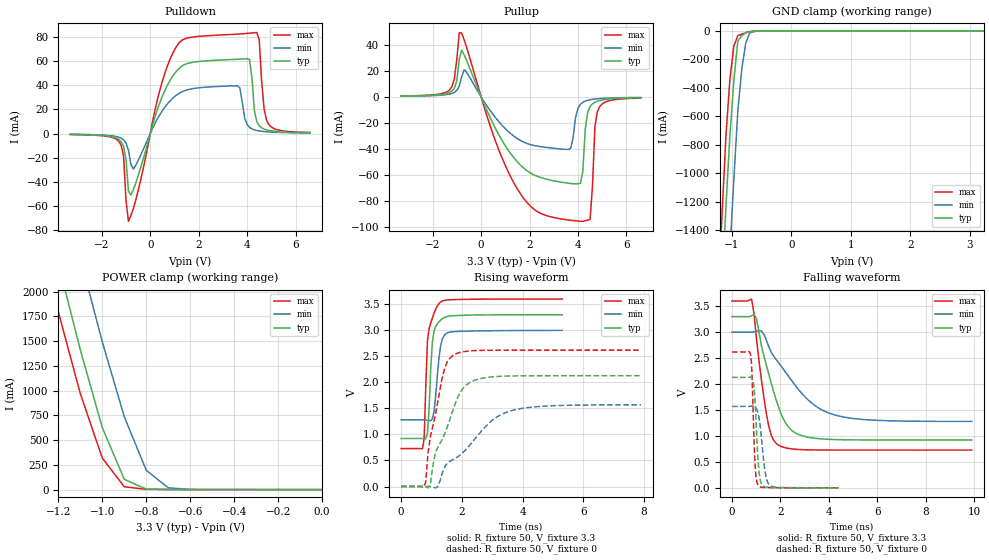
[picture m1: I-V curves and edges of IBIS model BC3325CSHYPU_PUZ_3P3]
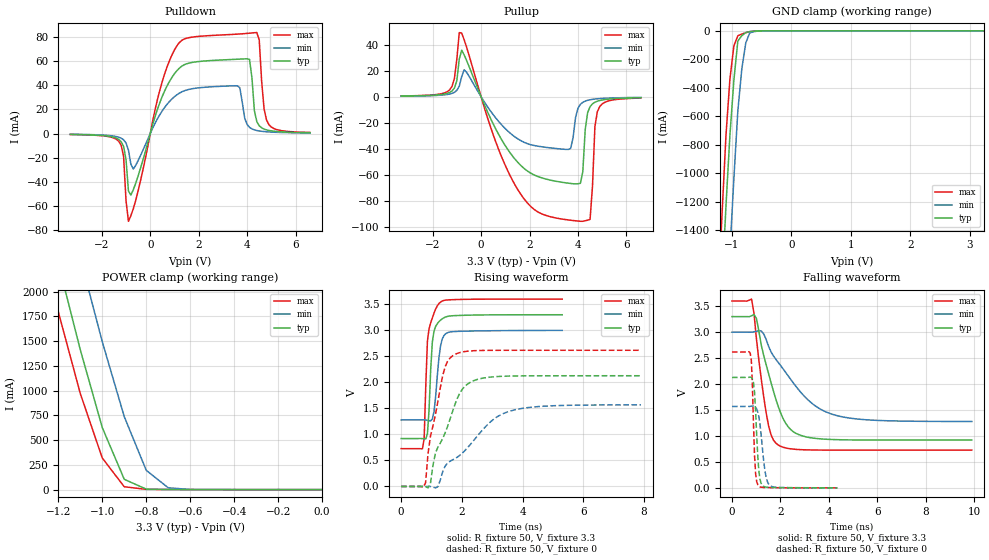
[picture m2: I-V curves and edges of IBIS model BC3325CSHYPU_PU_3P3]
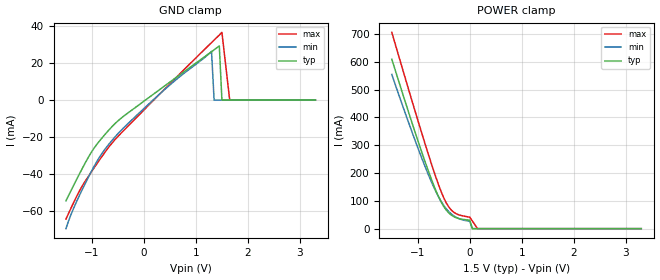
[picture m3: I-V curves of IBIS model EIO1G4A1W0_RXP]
[IBIS ver]   4.1
[File name]   xio3130_sandeer.ibs
[File Rev]   1.0
[Date]   September 10, 2007
[Source]   TI
[Notes]   Ver 1.1: Original September 10, 2007
| REV LOG:   1.0 original on August 21, 2006
|   Ver 1.1 is IBIS for PG 2.
[Disclaimer] Please be aware that in the absence of a written agreement
   Texas Instruments(TI) assumes no liability for: (1) The
   accuracy of the IBIS models provided to your company (2) The
   proper functioning of these Models in your design or for any
   resulting applications;or (3) Infringement of
   patents,copyrights or intellectual property rights resulting
   from your use of these models. TI provides IBIS Models as a
   service to our customers and therefore reserves the right to
   limit distribution of the Models.
[Copyright]   Property of Texas Instruments Incorporated. Unauthorised
   reproduction and/or distribution is strictly prohibited. This
   product is protected under copyright law and trade secret law
   as an unpublished work. Created 2007,(C) Copyright 2007,
   Texas Instruments Incorporated., All Rights Reserved. These
   commodities are under the U.S. Government distribution license
   control.As such,they are not to be re-exported without the
   prior approval of the U.S. Department of Commerce.
|   Component XIO3130
[Component]   XIO3130
[Manufacturer]   Texas Instruments.
[Package]
| variable   typ   min   max
R_pkg   2.09305e-001  8.11042e-003  5.46728e-001
L_pkg   3.90785e-009  1.26190e-009  1.07040e-008
C_pkg   1.04479e-012  5.09606e-013  6.63618e-012
[Pin]  signal_name   model_name  R_pin   L_pin   C_pin
A1 	PERST2		BC3325CSHYPU 	3.48182e-01	6.76130e-09	1.52376e-12
A12 	 PWR_GD0_GPIO2	BC3325CSHYPU 	3.39794e-01	4.78530e-09	6.39971e-13
A13 	VPP_1		POWER   2.77158e-01	4.95020e-09	1.35433e-12
A14	GPIO12		BC3325CSHYPU 	3.17830e-01	5.67010e-09	1.12048e-12
A2	PERST1		BC3325CSHYPU 	3.16708e-01	5.94340e-09	1.37649e-12
A6	DN_PERP_0	EIO1G4A1W0_RXP	3.07358e-01	4.42330e-09	9.38426e-13
A8	DN_PETP_0	EIO1G4A1W0_TX	3.02145e-01	4.33380e-09	1.15943e-12
A9	REFCKOP_0	 REFCLKOUT_C	3.39864e-01	4.83750e-09	9.84588e-13
B1 	PERST		IC33SFSHYPD	2.86998e-01	5.02970e-09	1.46470e-12
B11	PWR_ON0_GPIO1	BC3325CSHYPU 	2.96203e-01	3.82290e-09	6.38354e-13
B12	VPP_2		POWER   2.28630e-01	3.58240e-09	1.23695e-12
B13	GPIO13		BC3325CSHYPU 	2.56386e-01	4.03580e-09	1.36016e-12
B14	SCL		BC3325CSHYPU 	3.81111e-01	5.90920e-09	9.17494e-13
B5 	PERST0		BC3325CSHYPU 	2.52744e-01	3.39930e-09	9.88828e-13
B6	DN_PERN_0	EIO1G4A1W0_RXN	2.97653e-01	4.07660e-09	9.46291e-13
B8	DN_PETN_0	EIO1G4A1W0_TX	2.99772e-01	4.12360e-09	1.05127e-12
B9	REFCKON_0	REFCLKOUT_C	3.37041e-01	4.54020e-09	1.18566e-12
C10	DPSTRP0		BC3325CSHYPU 	1.67776e-01	2.10160e-09	8.80891e-13
C12	GPIO3		BC3325CSHYPU 	2.02085e-01	2.62660e-09	1.12832e-12
C2	GRST		IC33THYPU	2.55732e-01	3.73630e-09	1.72787e-12
C3	WAKE		BC3350BTOD	2.04369e-01	2.88420e-09	1.47207e-12
C4	VREG_EN   NC   1.72568e-01	2.16550e-09	1.53275e-12
C6	PRSNT0_GPIO0	BC3325CSHYPU 	1.59277e-01	2.01830e-09	1.29989e-12
D1	VSSDREF   GND   2.96673e-01	4.40840e-09	6.56277e-13
D13	SDA		BC3325CSHYPU 	3.10044e-01	4.05030e-09	8.29410e-13
D14	PRSNT1_GPIO4	BC3325CSHYPU 	2.72028e-01	4.51280e-09	8.91943e-13
D2	REFR0		NC   2.08243e-01	3.12100e-09	8.72610e-13
D4	TM_EN		IC33S   1.71885e-01	1.87770e-09	1.56170e-12
E1	VAUX33REF	POWER   2.95994e-01	4.32000e-09	5.85849e-13
E2	VDD33REF	POWER   2.58088e-01	3.37240e-09	7.27540e-13
E3	REFR1		NC   1.65373e-01	2.05030e-09	9.51770e-13
E4	VSSAREF	GND	1.71892e-01	1.87280e-09	1.13752e-12
F13	DN_PERP_1	EIO1G4A1W0_RXP	3.39229e-01	4.52580e-09	1.00466e-12
F14	DN_PERN_1	EIO1G4A1W0_RXP	3.40188e-01	4.70740e-09	8.48746e-13
F3	VDDAREF   POWER   1.96308e-01	2.26680e-09	1.07035e-12
G1	UP_PETP_1	EIO1G4A1W0_TX	2.92665e-01	4.25920e-09	7.86997e-13
G2	UP_PETN_1	EIO1G4A1W0_TX	2.89056e-01	4.03470e-09	9.71695e-13
H13	DN_PETP_1	EIO1G4A1W0_TX	2.91932e-01	3.96270e-09	8.44904e-13
H14	DN_PETN_1	EIO1G4A1W0_TX	2.91177e-01	4.24470e-09	8.54606e-13
J1 	 UP_PERP_1	EIO1G4A1W0_RXP	3.39760e-01	4.81770e-09	9.53436e-13
J14	REFCKON_1	REFCLKOUT_C	3.28820e-01	4.73900e-09	8.56505e-13
J2	 UP_PERN_1	EIO1G4A1W0_RXN	3.40049e-01	4.64620e-09	1.07197e-12
K14	REFCKOP_1	REFCLKOUT_C	3.31929e-01	4.68100e-09	6.52614e-13
L1	REFCKIP_1	PCIEREFIN_V30	3.97574e-01	6.00690e-09	1.41140e-12
L12	 PWR_ON1_GPIO5	BC3325CSHYPU 	1.85893e-01	2.41880e-09	1.02367e-12
L13	DPSTRP1		BC3325CSHYPU 	3.04921e-01	3.99150e-09	9.55643e-13
L2	REFCKIN_1	PCIEREFIN_V30	3.95837e-01	5.85920e-09	1.39246e-12
L3	GPIO18		BC3325CSHYPU 	2.29605e-01	3.05390e-09	1.35688e-12
M10	PRSNT2_GPIO8	BC3325CSHYPU 	1.74120e-01	2.17390e-09	1.07131e-12
M13	PWR_GD1_GPIO6	BC3325CSHYPU 	2.33053e-01	3.57840e-09	1.07590e-12
M14	GPIO15		BC3325CSHYPU 	2.77478e-01	4.66060e-09	8.47070e-13
M3	GPIO17_PWR_OVER	BC3325CSHYPU 	1.98049e-01	2.79690e-09	1.22160e-12
N11	GPIO11		BC3325CSHYPU 	2.23391e-01	3.27840e-09	8.83452e-13
N12	GPIO14		BC3325CSHYPU 	2.29447e-01	3.59270e-09	7.28550e-13
N2	CLKREQ_UP	BC3350BTOD	2.94360e-01	4.68110e-09	1.18772e-12
N3 	PWR_ON2_GPIO9	BC3325CSHYPU 	3.25542e-01	4.54360e-09	9.29756e-13
N4	DPSTRP2		BC3325CSHYPU 	3.06995e-01	4.01710e-09	7.83007e-13
N7	DN_PETP_2	EIO1G4A1W0_TX	2.90192e-01	3.96320e-09	9.35839e-13
N9	DN_PERP_2	EIO1G4A1W0_RXP	3.30597e-01	4.43580e-09	1.08021e-12
P1	REFCLK_SEL	IC33S   3.11848e-01	5.57690e-09	1.10777e-12
P12	GPIO16		BC3325CSHYPU 	3.48550e-01	4.99450e-09	8.65165e-13
P13	GPIO7		BC3325CSHYPU 	3.71036e-01	5.56470e-09	7.58018e-13
P2	PWR_GD2_GPIO10	BC3325CSHYPU 	2.86683e-01	5.10680e-09	1.31629e-12
P5	REFCKOP_2	 REFCLKOUT_C	3.43286e-01	4.84920e-09	5.90517e-13
P6	REFCKON_2	 REFCLKOUT_C	3.39679e-01	4.78910e-09	7.53869e-13
P7	DN_PETN_2	EIO1G4A1W0_TX	2.91402e-01	4.20940e-09	8.89549e-13
P9	DN_PERN_2	EIO1G4A1W0_RXN	3.35460e-01	4.62110e-09	9.64954e-13
[Model Selector]   BC3325CSHYPU
BC3325CSHYPU_PUZ_3P3  Cell operated at 3.3(nom) PULLUP_ON
BC3325CSHYPU_PU_3P3  Cell operated at 3.3(nom) PULLUP_OFF
[Model Selector]   IC33SFSHYPD
IC33SFSHYPD_3P3PD   Cell operated at VDDS=3.3V(typ) with pulldown "on"
IC33SFSHYPD_3P3PDZ   Cell operated at VDDS=3.3V(typ) with pulldown "off"
[Model Selector] IC33THYPU
IC33THYPU_3P3PU   Cell operated at VDDS=3.3V(nom) with Pullup "on"
IC33THYPU_3P3PUZ   Cell operated at VDDS=3.3V(nom) with Pullup "off"
[Model Selector]   IC33S
IC33S_2P5   Cell operated at VDDS=2.5V(nom)
IC33S_3P3   Cell operated at VDDS=3.3V(nom)
[Model] EIO1G4A1W0_TX
Model_type Output
Polarity Non-Inverting
Cref = 2.0pF
Rref = 50
Vref = 1.0V
Vmeas =1.0V
|   typ   min   max
C_comp   1.603pF   1.594pF   1.637pF
|[Model Spec]
[Driver Schedule]
| Model_name Rise_on_dly Rise_off_dly Fall_on_dly Fall_off_dly
high_high 0.0nS 0.4nS NA NA
medium_high 0.401nS 1.95nS NA NA
low_low NA NA 0.0nS 0.40nS
medium_low NA NA 0.401nS 2.05nS
[Temperature Range]   25   125   -40
[Voltage Range] 1.50V 1.35V 1.65V
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[Ramp]
| variable   typ   min   max
dV/dt_r 1V/0.001ns  0.21654V/0.0277367ns  0.198V/0.0212173ns
dV/dt_f 1V/0.001ns  0.21654V/0.0277367ns  0.198V/0.0212173ns
R_load = 50
| Models and submodels in the file (18): BC3325CSHYPU_PUZ_3P3 (I/O), BC3325CSHYPU_PU_3P3 (I/O), EIO1G4A1W0_RXP (Input), EIO1G4A1W0_RXN (Input), REFCLKOUT_C (Output), IC33SFSHYPD_3P3PD (Input), IC33SFSHYPD_3P3PDZ (Input), EIO1G4A1W0_TX (Output), high_high (Open_source), low_low (Open_drain), medium_high (Open_source), medium_low (Open_drain), IC33THYPU_3P3PU (Input), IC33THYPU_3P3PUZ (Input), BC3350BTOD (I/O_open_drain), IC33S_2P5 (Input), IC33S_3P3 (Input), PCIEREFIN_V30 (Input)
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|   Model Cell BC3325CSHYPU_PUZ_3P3
[Model]   BC3325CSHYPU_PUZ_3P3
Model_type   I/O
Polarity   Non-Inverting
Enable   Active-Low
Vinl =  0.8v
Vinh =  2v
Cref =  15.0000pF
Rref =  100.0000M
Vref =  0V
Vmeas =  1.65
C_comp   2.096801p   2.080601p   2.168299p
[Model Spec]
Vinl   0.8v   0.8V   0.8V
Vinh   2v   2V   2V
[Temperature Range]   25   125   -40
[Voltage Range]   3.3   3   3.6
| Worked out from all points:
|   slope of the pulldown table from 0 to 0.495 V, typ, clamps not added: 16.1 ohm
|   slope of the pullup table from 0 to 0.495 V, typ, clamps not added: 23.9 ohm
|   GND clamp passes 1 mA (typ) near -0.57 V on its own axis
|   POWER clamp passes 1 mA (typ) near -0.70 V on its own axis
|   rising waveform, R_fixture 50, V_fixture 3.3: 20-80 % time 131ps typ, 171ps min, 141ps max; typ from 0.923 V to 3.3 V
|   rising waveform, R_fixture 50, V_fixture 0: 20-80 % time 804ps typ, 1.58ns min, 487ps max; typ from 0.001 V to 2.13 V
|   falling waveform, R_fixture 50, V_fixture 3.3: 20-80 % time 871ps typ, 1.74ns min, 492ps max; typ from 3.3 V to 0.923 V
|   falling waveform, R_fixture 50, V_fixture 0: 20-80 % time 145ps typ, 222ps min, 111ps max; typ from 2.13 V to 0.001 V
[POWER_clamp]
|   voltage   I(typ)   I(min)   I(max)
-3.3V     22.69A     23.55A     22.21A
-1.233V   2.591A     3.534A     2.093A
-1.2V     2.287A     3.229A     1.795A
-1.167V   1.995A     2.933A     1.52A
-1.1V     1.413A     2.34A      970.4mA
-1.067V   1.151A     2.058A     753.2mA
-1.033V   888.5mA    1.776A     536.1mA
-1V       626.4mA    1.494A     318.9mA
-900mV    104mA      736.8mA    28.83mA
-800mV    4.946mA    194.9mA    2.696mA
-700mV    998.1uA    18.43mA    1.144mA
-11.55fV  218.9pA    3.023nA    211.8pA
[Pulldown]
|   voltage   I(typ)   I(min)   I(max)
-3.3V     -705.5uA   -563.9uA   -760.4uA
-1.3V     -4.855mA   -3.026mA   -6.366mA
-1.1V     -10.66mA   -5.175mA   -19.03mA
-900mV    -47.6mA    -13.63mA   -72.85mA
-700mV    -46.65mA   -29.39mA   -62.46mA
1.1V      52.19mA    32.2mA     72.89mA
3.6V      61.75mA    39.68mA    82.61mA
4.1V      61.59mA    5.155mA    83.39mA
4.4V      9.95mA     2.546mA    83.89mA
4.7V      3.744mA    1.667mA    20.57mA
4.9V      2.605mA    1.352mA    7.423mA
6.6V      709.5uA    512.8uA    930uA
[Pullup]
|   voltage   I(typ)   I(min)   I(max)
-3.3V     505.9uA    408uA      584.9uA
-1.3V     3.261mA    2.062mA    5.225mA
-800mV    35.78mA    15.51mA    48.94mA
600mV     -24.59mA   -16.18mA   -34.36mA
1.6V      -52.1mA    -33.35mA   -73.91mA
3.7V      -66.73mA   -39.75mA   -95mA
4.2V      -57.72mA   -4.291mA   -95.81mA
4.3V      -25.25mA   -3.364mA   -95.38mA
4.5V      -7.634mA   -2.331mA   -94.34mA
4.7V      -4.24mA    -1.775mA   -22.94mA
4.9V      -2.904mA   -1.43mA    -7.534mA
6.6V      -771.5uA   -533.2uA   -1.015mA
[GND_clamp]
|   voltage   I(typ)   I(min)   I(max)
-3.3V     -22.48A    -23.28A    -22.04A
-1.233V   -2.398A    -3.286A    -1.879A
-1.167V   -1.809A    -2.69A     -1.297A
-1.1V     -1.235A    -2.104A    -738.1mA
-1.033V   -735.2mA   -1.553A    -340.6mA
-966.7mV  -347.6mA   -1.039A    -106.1mA
-900mV    -71.93mA   -563.2mA   -34.66mA
-833.3mV  -34.38mA   -267.8mA   -23.1mA
-766.7mV  -12.31mA   -84.87mA   -13.47mA
-700mV    -5.7mA     -14.32mA   -5.752mA
-500mV    -215.1uA   -473.8uA   -210uA
3.233V    -4.928uA   12.61uA    -38.06uA
[Ramp]
| variable   typ   min   max
dV/dt_r   1.29409/0.8072212n  0.9574059/1.586115n   1.586195/0.4872986n
dV/dt_f   1.451701/0.8772609n   1.051893/1.749039n   1.750196/0.494297n
R_load = 50
[Rising Waveform]
R_fixture = 50
V_fixture = 3.3
V_fixture_min = 3
V_fixture_max = 3.6
|   time   V(typ)   V(min)   V(max)
0s        922.7mV    1.28V      729.2mV
703ps     921.8mV    1.281V     727mV
758ps     915.9mV    1.281V     919.8mV
866ps     1.014V     1.274V     2.793V
920ps     1.476V     1.265V     3.029V
1.028ns   2.771V     1.3V       3.237V
1.083ns   2.982V     1.438V     3.33V
1.299ns   3.196V     2.699V     3.544V
1.624ns   3.277V     2.968V     3.587V
5.308ns   3.3V       2.999V     3.6V
[Rising Waveform]
R_fixture = 50
V_fixture = 0
V_fixture_min = 0
V_fixture_max = 0
|   time   V(typ)   V(min)   V(max)
0s        1.034mV    901.2uV    1.259mV
805ps     -3.192mV   1.663mV    73.26mV
886ps     -25.74mV   2.498mV    638.9mV
966ps     62.2mV     -720.8uV   971.7mV
1.127ns   640.5mV    -25.36mV   1.378V
1.369ns   925.5mV    285.7mV    2.132V
1.772ns   1.576V     537.9mV    2.539V
2.336ns   2.02V      847.5mV    2.608V
3.545ns   2.123V     1.443V     2.618V
7.9ns     2.129V     1.569V     2.619V
[Falling Waveform]
R_fixture = 50
V_fixture = 3.3
V_fixture_min = 3
V_fixture_max = 3.6
|   time   V(typ)   V(min)   V(max)
0s        3.3V       3V         3.6V
807ps     3.315V     2.999V     3.636V
908ps     3.342V     3.006V     3.368V
1.009ns   3.263V     3.016V     2.878V
1.413ns   2.374V     2.857V     1.447V
1.615ns   2.028V     2.619V     1.024V
1.918ns   1.562V     2.414V     825.2mV
2.625ns   1.057V     1.967V     744.6mV
4.241ns   931.8mV    1.405V     729.5mV
9.896ns   922.7mV    1.281V     729.2mV
[Falling Waveform]
R_fixture = 50
V_fixture = 0
V_fixture_min = 0
V_fixture_max = 0
|   time   V(typ)   V(min)   V(max)
0s        2.129V     1.57V      2.619V
762ps     2.136V     1.573V     2.583V
806ps     2.127V     1.577V     2.41V
941ps     1.776V     1.566V     533.5mV
986ps     1.372V     1.544V     232.8mV
1.076ns   528.8mV    1.446V     54mV
1.21ns    83.11mV    993mV      14.02mV
1.39ns    17.89mV    250.3mV    8.278mV
1.569ns   9.376mV    45.86mV    6.2mV
4.396ns   1.208mV    1.902mV    1.277mV
|   Model Cell BC3325CSHYPU_PU_3P3
[Model]   BC3325CSHYPU_PU_3P3
Model_type   I/O
Polarity   Non-Inverting
Enable   Active-Low
Vinl =  0.8v
Vinh =  2v
Cref =  15.0000pF
Rref =  100.0000M
Vref =  0V
Vmeas =  1.65
C_comp   2.096801p   2.080601p   2.168299p
[Model Spec]
Vinl   0.8v   0.8V   0.8V
Vinh   2v   2V   2V
[Temperature Range]   25   125   -40
[Voltage Range]   3.3   3   3.6
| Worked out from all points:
|   slope of the pulldown table from 0 to 0.495 V, typ, clamps not added: 16.1 ohm
|   slope of the pullup table from 0 to 0.495 V, typ, clamps not added: 23.9 ohm
|   GND clamp passes 1 mA (typ) near -0.57 V on its own axis
|   POWER clamp passes 1 mA (typ) near -0.70 V on its own axis
|   rising waveform, R_fixture 50, V_fixture 3.3: 20-80 % time 130ps typ, 170ps min, 140ps max; typ from 0.921 V to 3.3 V
|   rising waveform, R_fixture 50, V_fixture 0: 20-80 % time 804ps typ, 1.58ns min, 487ps max; typ from 0 V to 2.13 V
|   falling waveform, R_fixture 50, V_fixture 3.3: 20-80 % time 869ps typ, 1.74ns min, 491ps max; typ from 3.3 V to 0.921 V
|   falling waveform, R_fixture 50, V_fixture 0: 20-80 % time 146ps typ, 220ps min, 112ps max; typ from 2.13 V to 0 V
[POWER_clamp]
|   voltage   I(typ)   I(min)   I(max)
-3.3V     22.69A     23.55A     22.21A
-1.233V   2.591A     3.534A     2.093A
-1.2V     2.287A     3.229A     1.795A
-1.167V   1.995A     2.933A     1.52A
-1.1V     1.413A     2.34A      970.4mA
-1.067V   1.151A     2.058A     753.2mA
-1.033V   888.5mA    1.776A     536.1mA
-1V       626.4mA    1.494A     318.9mA
-900mV    104mA      736.8mA    28.76mA
-800mV    4.906mA    194.9mA    2.602mA
-700mV    943.7uA    18.42mA    1.061mA
-11.55fV  219.4pA    3.023nA    212.4pA
[Pulldown]
|   voltage   I(typ)   I(min)   I(max)
-3.3V     -705.5uA   -563.9uA   -760.4uA
-1.3V     -4.855mA   -3.026mA   -6.366mA
-1.1V     -10.66mA   -5.175mA   -19.03mA
-900mV    -47.6mA    -13.63mA   -72.85mA
-700mV    -46.65mA   -29.39mA   -62.46mA
1.1V      52.19mA    32.2mA     72.89mA
3.6V      61.75mA    39.68mA    82.61mA
4.1V      61.59mA    5.155mA    83.39mA
4.4V      9.95mA     2.546mA    83.89mA
4.7V      3.744mA    1.667mA    20.57mA
4.9V      2.605mA    1.352mA    7.423mA
6.6V      709.5uA    512.8uA    930uA
[Pullup]
|   voltage   I(typ)   I(min)   I(max)
-3.3V     505.9uA    408uA      584.9uA
-1.3V     3.261mA    2.062mA    5.225mA
-800mV    35.78mA    15.51mA    48.94mA
600mV     -24.59mA   -16.18mA   -34.36mA
1.6V      -52.1mA    -33.35mA   -73.91mA
3.7V      -66.73mA   -39.75mA   -95mA
4.2V      -57.72mA   -4.291mA   -95.81mA
4.3V      -25.25mA   -3.364mA   -95.38mA
4.5V      -7.633mA   -2.331mA   -94.34mA
4.7V      -4.24mA    -1.775mA   -22.93mA
4.9V      -2.904mA   -1.43mA    -7.534mA
6.6V      -771.5uA   -533.2uA   -1.015mA
[GND_clamp]
|   voltage   I(typ)   I(min)   I(max)
-3.3V     -22.48A    -23.28A    -22.04A
-1.233V   -2.398A    -3.286A    -1.879A
-1.167V   -1.809A    -2.69A     -1.297A
-1.1V     -1.235A    -2.104A    -738mA
-1.033V   -735.2mA   -1.553A    -340.5mA
-966.7mV  -347.6mA   -1.039A    -106mA
-900mV    -71.85mA   -563.2mA   -34.5mA
-833.3mV  -34.29mA   -267.8mA   -22.94mA
-766.7mV  -12.21mA   -84.82mA   -13.3mA
-700mV    -5.6mA     -14.26mA   -5.59mA
-433.3mV  -42.37uA   -170.9uA   -16.21uA
3.233V    209.8pA    805.5nA    182.4pA
[Ramp]
| variable   typ   min   max
dV/dt_r   1.293947/0.8069069n  0.9572319/1.586102n   1.586179/0.4868774n
dV/dt_f   1.453004/0.8754339n   1.053061/1.747481n   1.751657/0.4923244n
R_load = 50
[Rising Waveform]
R_fixture = 50
V_fixture = 3.3
V_fixture_min = 3
V_fixture_max = 3.6
|   time   V(typ)   V(min)   V(max)
0s        920.7mV    1.278V     727mV
703ps     919.9mV    1.279V     724.7mV
758ps     913.9mV    1.279V     916.7mV
866ps     1.012V     1.272V     2.796V
920ps     1.474V     1.263V     3.031V
1.028ns   2.775V     1.298V     3.238V
1.083ns   2.986V     1.436V     3.331V
1.299ns   3.197V     2.703V     3.545V
1.624ns   3.277V     2.97V      3.587V
5.308ns   3.3V       2.999V     3.6V
[Rising Waveform]
R_fixture = 50
V_fixture = 0
V_fixture_min = 0
V_fixture_max = 0
|   time   V(typ)   V(min)   V(max)
0s        1.388nV    41.17nV    487.2pV
805ps     -4.225mV   761.8uV    70.6mV
886ps     -26.93mV   1.601mV    633.1mV
966ps     59.91mV    -1.616mV   965.2mV
1.128ns   638.3mV    -26.44mV   1.376V
1.37ns    922.6mV    284.8mV    2.133V
1.773ns   1.575V     535.4mV    2.538V
2.337ns   2.019V     845.7mV    2.607V
3.546ns   2.121V     1.441V     2.617V
7.902ns   2.128V     1.568V     2.617V
[Falling Waveform]
R_fixture = 50
V_fixture = 3.3
V_fixture_min = 3
V_fixture_max = 3.6
|   time   V(typ)   V(min)   V(max)
0s        3.3V       3V         3.6V
807ps     3.315V     2.999V     3.637V
908ps     3.342V     3.006V     3.366V
1.009ns   3.263V     3.017V     2.87V
1.412ns   2.37V      2.858V     1.44V
1.614ns   2.024V     2.617V     1.02V
1.917ns   1.558V     2.412V     822.5mV
2.624ns   1.054V     1.965V     742.3mV
4.239ns   929.9mV    1.403V     727.3mV
9.893ns   920.7mV    1.279V     727mV
[Falling Waveform]
R_fixture = 50
V_fixture = 0
V_fixture_min = 0
V_fixture_max = 0
|   time   V(typ)   V(min)   V(max)
0s        2.128V     1.569V     2.617V
753ps     2.135V     1.571V     2.595V
798ps     2.129V     1.575V     2.459V
886ps     2.029V     1.576V     1.248V
975ps     1.476V     1.549V     274.8mV
1.108ns   333mV      1.376V     31.31mV
1.197ns   93.8mV     1.05V      12.91mV
1.374ns   17.46mV    288.9mV    6.924mV
1.552ns   8.127mV    50.33mV    4.931mV
4.345ns   182.2uV    1.001mV    19.76uV
|   Model EIO1G4A1W0_RXP
[Model]   EIO1G4A1W0_RXP
Model_type   Input
Polarity   Non-Inverting
Vinl =  -0.6000V
Vinh =   0.6000V
C_comp   1.6030pF   1.5940pF   1.6370pF
[Temperature Range]   25.0000   0.1250k   -40.0000
[Voltage Range]   1.5000V   1.3500V   1.6500V
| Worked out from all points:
|   GND clamp passes 1 mA (typ) near -0.02 V on its own axis
[GND_clamp]
| voltage   I(typ)   I(min)   I(max)
-1.5V     -54.27mA   -69.3mA    -64.12mA
-1.35V    -45.8mA    -58.06mA   -55.04mA
-1.15V    -34.9mA    -46.09mA   -44.62mA
-750mV    -18.53mA   -26.47mA   -28.1mA
-450mV    -9.994mA   -16.62mA   -18.12mA
650mV     12.8mA     11.72mA    13.03mA
1.3V      26.07mA    26.24mA    30.98mA
1.35V     27.09mA    0A         32.34mA
1.45V     29.19mA    0A         35.08mA
1.5V      0A         0A         36.49mA
1.65V     0A         0A         0A
3.3V      0A         0A         0A
[POWER_clamp]
| voltage   I(typ)   I(min)   I(max)
-1.5V     609.2mA    554.5mA    705.6mA
-1.05V    345.7mA    316.2mA    421.1mA
-850mV    235.3mA    218.6mA    298.9mA
-700mV    159mA      152.5mA    211.5mA
-600mV    114.5mA    114.2mA    157.4mA
-500mV    79.22mA    83.16mA    110.5mA
-400mV    55.87mA    60.42mA    76.74mA
-300mV    42.38mA    45.06mA    57.86mA
0V        30.28mA    26.63mA    41.13mA
50mV      0A         0A         27.42mA
150mV     0A         0A         0A
3.3V      0A         0A         0A
